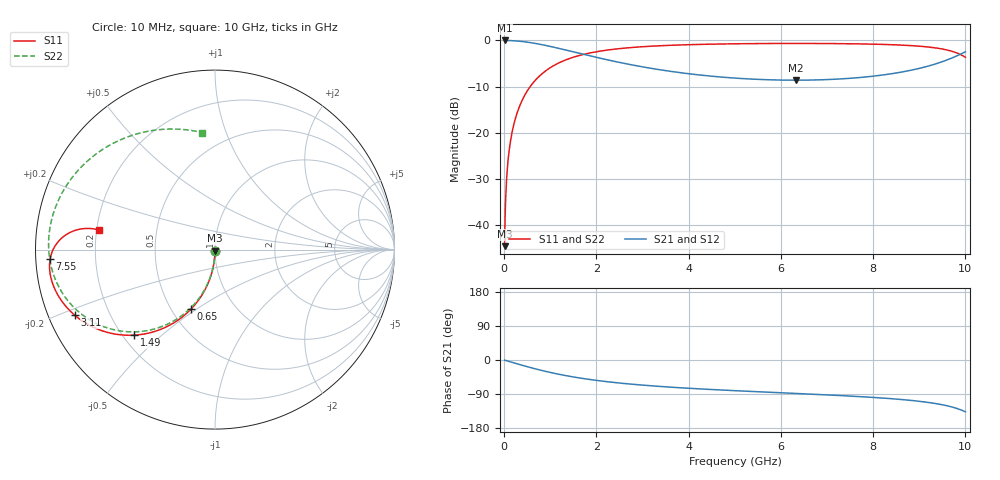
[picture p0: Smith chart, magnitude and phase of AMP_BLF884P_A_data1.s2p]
! Created Thu Nov 14 15:30:41 2013
# ghz S ma R 50
! 2 Port Network Data from SP1.SP block
! freq  magS11  angS11  magS21  angS21  magS12  angS12  magS22  angS22
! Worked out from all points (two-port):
!   1000 points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, 10 MHz to 10 GHz, reference 50 ohm
!   highest |S21| = 0.00 dB at 10 MHz (marker M1); lowest = -8.6 dB at 6.32 GHz (marker M2)
!   |S21| within 3 dB of the highest: start of sweep to 1.72 GHz; 9.888 GHz to end of sweep
!   lowest |S11| = -44.6 dB at 10 MHz (marker M3), VSWR 1.01, Z = 50 - j0.592 ohm
!   |S11| at or under -10 dB: start of sweep to 563.8 MHz
!   |S22| runs from -44.6 to -0.6 dB; largest |S21 - S12| = 0
!   S11 on the Smith chart (normalised r, x): 10 MHz: 1.00, -0.01; 650 MHz: 0.62, -0.48; 1.49 GHz: 0.24, -0.41; 3.11 GHz: 0.08, -0.22; 7.55 GHz: 0.04, -0.03; 10 GHz: 0.21, +0.08
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0.01  0.005921 -90.3  1 -0.4  1 -0.4  0.005921 -90.4
0.07  0.04142 -92.5  0.9991 -2.5  0.9991 -2.5  0.04142 -92.6
0.09  0.05322 -93.2  0.9986 -3.3  0.9986 -3.3  0.05322 -93.3
0.13  0.07676 -94.6  0.997 -4.7  0.997 -4.7  0.07676 -94.8
0.19  0.1118 -96.7  0.9937 -6.9  0.9937 -6.9  0.1118 -97.0
0.37  0.2139 -102.9  0.9768 -13.2  0.9768 -13.2  0.2139 -103.5
0.65  0.3585 -112.0  0.9335 -22.5  0.9335 -22.5  0.3585 -113.0
1.01  0.5109 -122.3  0.8596 -33.1  0.8596 -33.1  0.5109 -123.9
1.49  0.656 -133.4  0.7548 -44.5  0.7548 -44.5  0.6559 -135.7
1.68  0.6982 -137.0  0.7159 -48.3  0.7159 -48.3  0.6982 -139.6
2.34  0.7991 -146.9  0.6012 -58.7  0.6012 -58.7  0.7991 -150.6
3.11  0.8623 -154.9  0.5064 -67.4  0.5064 -67.4  0.8622 -159.8
3.34  0.8746 -156.7  0.4848 -69.4  0.4848 -69.4  0.8745 -162.1
5.01  0.9204 -166.6  0.3909 -81.0  0.3909 -81.0  0.9203 -175.4
6.32  0.9285 -172.0  0.3713 -88.2  0.3713 -88.2  0.9284 175.5
6.67  0.9279 -173.3  0.3727 -90.2  0.3727 -90.2  0.9278 173.0
7.55  0.9204 -176.7  0.3909 -95.5  0.3909 -95.5  0.9202 165.7
8.34  0.9019 180.0  0.4317 -101.6  0.4317 -101.6  0.9018 156.9
8.94  0.8714 176.8  0.4903 -108.1  0.4903 -108.1  0.8712 146.9
9.38  0.8267 173.9  0.5624 -115.4  0.5624 -115.4  0.8264 135.3
9.7  0.7654 171.5  0.6433 -123.7  0.6433 -123.7  0.765 121.1
10  0.6568 170.4  0.7537 -136.7  0.7537 -136.7  0.6561 96.3
